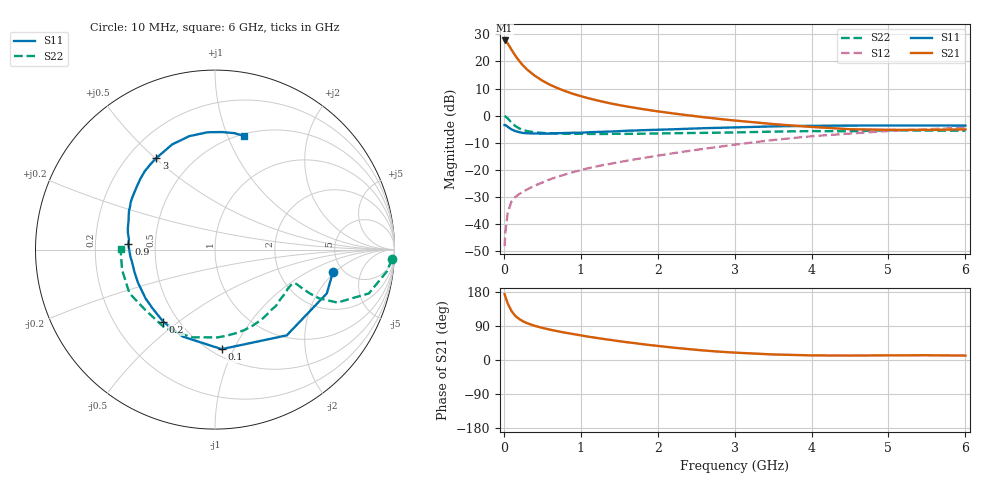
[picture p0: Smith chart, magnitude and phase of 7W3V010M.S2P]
! Infineon Technologies  Discrete & RF Semiconductors
! BFS17W
! Si NPN RF Bipolar Junction Transistor in SOT323
! VCE = 3 V  IC = 10 mA
! Common Emitter S-Parameters:  August  1999
# GHz  S  MA  R  50
!  f  S11  S21  S12  S22
! GHz  MAG  ANG  MAG  ANG  MAG  ANG  MAG  ANG
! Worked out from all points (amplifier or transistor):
!   36 points, 10 MHz to 6 GHz, reference 50 ohm
!   highest |S21| = 27.7 dB at 10 MHz (marker M1)
!   |S21| within 3 dB of that: start of sweep to 91.25 MHz
!   unconditionally stable (mu >= 1): 393.2 MHz to 2.562 GHz; 4.386 GHz to end of sweep
!   at 250 MHz: K = 0.80, MSG = 23.3 dB, |S12| = -28.1 dB
!   at 1.4 GHz: K = 1.22, MAG = 8.3 dB, |S12| = -17.7 dB
!   at 6 GHz: K = 1.07, MAG = -1.9 dB, |S12| = -4.5 dB
!   S11 on the Smith chart (normalised r, x): 10 MHz: 4.17, -1.86; 100 MHz: 0.56, -0.90; 200 MHz: 0.41, -0.44; 900 MHz: 0.35, +0.03; 3 GHz: 0.31, +0.50; 6 GHz: 0.52, +1.15
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0.01  0.6691 -10.6  24.35 173.8  0.0039 82.1  0.9864 -3.1
0.02  0.6691 -21.4  23.94 166.9  0.0071 81.8  0.9666 -7.1
0.05  0.623 -50.1  21.48 149.3  0.0161 69.0  0.8915 -15.9
0.1  0.5558 -86.2  16.45 129.1  0.0262 58.3  0.7428 -23.4
0.15  0.5169 -110.4  12.7 116.2  0.0316 52.9  0.6403 -25.1
0.2  0.4949 -125.6  10.17 108.1  0.0357 53.5  0.5806 -24.8
0.25  0.4776 -136.8  8.398 102.0  0.0393 53.5  0.5421 -24.1
0.3  0.473 -144.9  7.133 97.4  0.0432 54.8  0.5198 -23.6
0.4  0.467 -156.9  5.468 90.2  0.051 57.3  0.4919 -22.9
0.5  0.4659 -164.7  4.423 84.8  0.0581 59.7  0.4796 -23.0
0.6  0.4665 -170.4  3.703 80.1  0.0667 61.3  0.4715 -23.8
0.7  0.473 -175.4  3.207 75.9  0.0748 62.8  0.4663 -25.2
0.9  0.483 176.5  2.519 68.5  0.0905 64.7  0.4599 -28.7
1.1  0.4928 169.6  2.09 61.5  0.1072 65.5  0.4595 -33.1
1.3  0.5043 163.4  1.787 55.4  0.1231 66.1  0.4577 -38.1
1.6  0.5263 155.5  1.472 46.9  0.1471 66.9  0.4599 -45.9
2.2  0.559 141.3  1.098 32.7  0.202 67.4  0.4731 -63.6
3  0.6056 122.7  0.812 19.5  0.2909 64.3  0.4895 -88.5
3.5  0.6326 112.2  0.698 14.6  0.3544 59.9  0.5059 -105.0
4.5  0.6549 93.7  0.561 11.7  0.4663 47.5  0.5135 -138.7
5.5  0.6577 80.6  0.544 12.5  0.5607 35.0  0.5299 -167.7
6  0.6538 75.5  0.557 11.7  0.5972 28.9  0.5264 179.5
